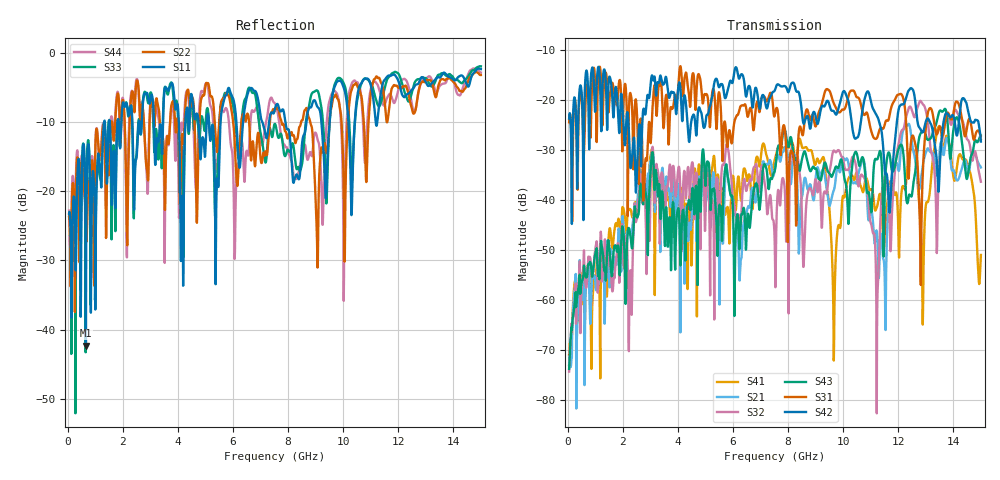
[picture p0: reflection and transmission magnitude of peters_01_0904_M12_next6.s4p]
# MHZ S RI R 50.00
! FREQ  S11  S12  S13  S14
!  S21  S22  S23  S24
!  S31  S32  S33  S34
!  S41  S42  S43  S44
!  REAL  IMAG  REAL  IMAG  REAL  IMAG  REAL  IMAG
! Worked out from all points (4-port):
!   1496 points, 50 MHz to 15 GHz, reference 50 ohm
!   strongest paths, dB at 50 MHz, 3.79 GHz, 7.53 GHz, 11.27 GHz, 15 GHz:
!     S42: -23.8, -18.5, -18.0, -23.7, -28.3
!     S31: -24.5, -21.8, -22.7, -26.9, -27.8
!     S43: -73.7, -43.5, -33.8, -31.5, -27.2
!     S32: -74.3, -34.8, -53.6, -55.8, -36.4
!     S21: -73.1, -36.7, -33.6, -52.0, -33.5
!     S41: -70.9, -39.0, -31.7, -40.3, -51.0
!   lowest |S11| = -42.3 dB at 660 MHz (marker M1), VSWR 1.02, Z = 50.5 + j0.617 ohm
!   |S11| at or under -10 dB: start of sweep to 1.322 GHz; 5.125 GHz to 5.549 GHz (423.5 MHz wide, 7.94 % of centre); 7.901 GHz to 8.667 GHz (765.7 MHz wide, 9.24 % of centre)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
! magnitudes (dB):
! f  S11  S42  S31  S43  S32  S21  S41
! 50 MHz  -23.3  -23.8  -24.5  -73.7  -74.3  -73.1  -70.9
! 660 MHz  -42.3  -14.6  -18.9  -55.4  -57.4  -56.8  -56.9
! 9.81 GHz  -4.1  -22.1  -22.3  -33.6  -30.1  -33.6  -45.5
! 11.24 GHz  -10.0  -23.4  -27.5  -31.9  -60.4  -47.5  -41.1
! 12.88 GHz  -3.6  -26.5  -36.3  -26.4  -20.8  -33.6  -59.5
! 13.48 GHz  -3.6  -37.2  -25.6  -22.5  -33.9  -31.9  -25.3
! 15 GHz  -2.4  -28.3  -27.8  -27.2  -36.4  -33.5  -51.0
